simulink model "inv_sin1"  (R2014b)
settings: Solver=ode45  StartTime=0.0  StopTime=10.0  RelTol=1e-3
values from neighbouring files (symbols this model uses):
  delta = nord/2    (= 32)    [hilbert_filter_1.m]    (also in hilbert_filter_2.m; hilbert_filter_3.m; inv_sinc_1.m = 25; komplexe_huelle_1.m)
  h = firls(n, f, a, wi)    [fir_ls_1.m]    (also in fir_pm_2.m = firpm(n, f0, a0, wi); fir_pm_3.m = firpm(n, f0, a0, wi); ideale_filter_4.m = fir1(N, [fs1, fs2]*2/fs, 'stop', hamming(N+1)); inv_sinc_1.m = hd)
  Ts = 1/fs    (= 0.001)    [abtast_fir_1.m]    (also in abtast_fir_2.m; abtast_fir_3.m; abtast_fir_4.m; hilbert_filter_1.m)

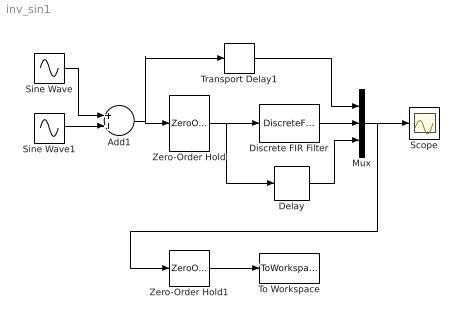
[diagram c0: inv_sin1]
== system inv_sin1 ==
  Add1 : Sum
  Delay : Delay  DelayLength=delta
  Discrete FIR Filter : DiscreteFir  Coefficients=h
  Mux : Mux  Inputs=3
  Scope : Scope
  Sine Wave : Sin  Frequency=2*pi*100  SampleTime=0
  Sine Wave1 : Sin  Frequency=2*pi*350  SampleTime=0
  To Workspace : ToWorkspace  VariableName=y  SaveFormat=Timeseries  SampleTime=-1
  Transport Delay1 : TransportDelay  DelayTime=Ts*delta
  Zero-Order Hold : ZeroOrderHold  SampleTime=Ts
  Zero-Order Hold1 : ZeroOrderHold  SampleTime=0.1*Ts
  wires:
  Mux/1 -> Scope/1, Zero-Order Hold1/1
  Add1/1 -> Transport Delay1/1, Zero-Order Hold/1
  Transport Delay1/1 -> Mux/1
  Zero-Order Hold/1 -> Delay/1, Discrete FIR Filter/1
  Delay/1 -> Mux/3
  Sine Wave/1 -> Add1/1
  Sine Wave1/1 -> Add1/2
  Discrete FIR Filter/1 -> Mux/2
  Zero-Order Hold1/1 -> To Workspace/1
